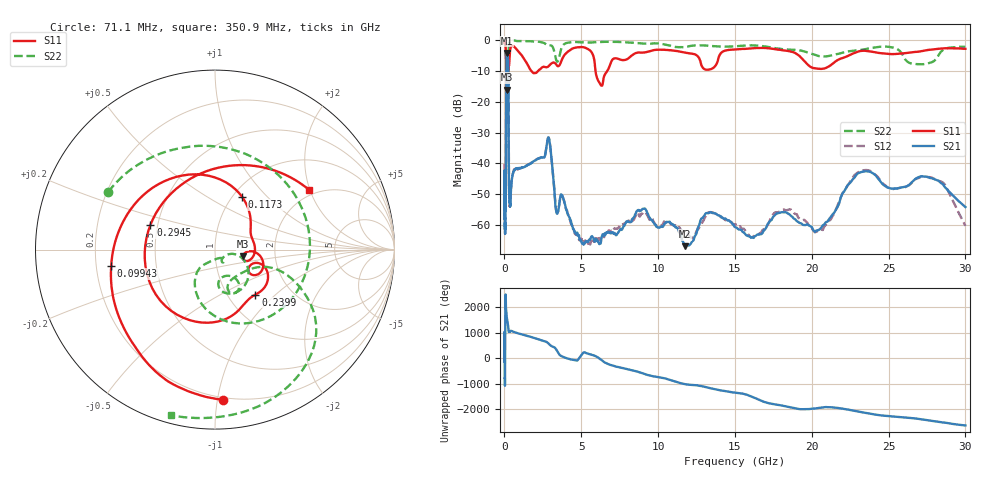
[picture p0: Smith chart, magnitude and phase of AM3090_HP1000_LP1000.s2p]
! Date/Time: Thu, Feb 28, 2019 2:02 PM
! Network Analyzer: Agilent Technologies E8364B Rev: A.07.50.67
! Sweep from 0.010 to 30.000 GHz, 1601 Points, Sweep Type: LOG
! Power Supply: 5.023 V, 0.002 A
# Hz S DB R 50
!freq MagS11 AngS11 MagS21 AngS21 MagS12 AngS12 MagS22 AngS22
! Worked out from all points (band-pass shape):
!   1601 points, 10 MHz to 30 GHz, reference 50 ohm
!   highest |S21| = -4.20 dB at 159.9 MHz (marker M1); lowest = -66.9 dB at 11.77 GHz (marker M2)
!   |S21| within 3 dB of the highest: 122.3 MHz to 242.5 MHz (120.2 MHz wide, 65.9 % of centre)
!   lowest |S11| = -16.0 dB at 152.9 MHz (marker M3), VSWR 1.37, Z = 67.9 - j5.19 ohm
!   |S11| at or under -10 dB: 118 MHz to 223 MHz (105 MHz wide, 61.6 % of centre); 1.745 GHz to 2.193 GHz (447.8 MHz wide, 22.7 % of centre); 5.925 GHz to 6.695 GHz (770.7 MHz wide, 12.2 % of centre)
!   |S22| runs from -25.7 to -0.1 dB; largest |S21 - S12| = 0.0097
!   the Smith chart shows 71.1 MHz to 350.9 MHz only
!   S11 on the Smith chart (normalised r, x): 71.1 MHz: 0.19, -1.04; 99.43 MHz: 0.26, -0.07; 117.3 MHz: 1.10, +0.73; 239.9 MHz: 1.34, -0.76; 294.5 MHz: 0.46, +0.15; 350.9 MHz: 1.83, +1.98
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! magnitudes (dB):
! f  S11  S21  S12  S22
! 10 MHz  -0.2  -42.4  -40.2  -0.6
! 38.04 MHz  -0.5  -59.0  -58.6  -1.5
! 71.1 MHz  -1.5  -54.5  -52.4  -3.4
! 86.86 MHz  -2.8  -53.2  -51.8  -4.9
! 99.43 MHz  -4.7  -33.7  -33.8  -5.5
! 117.3 MHz  -9.6  -10.1  -10.1  -12.5
! 144.7 MHz  -14.6  -4.4  -4.4  -23.9
! 152.9 MHz  -16.0  -4.2  -4.2  -21.3
! 159.9 MHz  -14.9  -4.2  -4.1  -16.6
! 239.9 MHz  -9.4  -6.9  -6.8  -13.5
! 294.5 MHz  -8.3  -48.1  -47.8  -1.2
! 350.9 MHz  -4.1  -52.7  -53.9  -0.4
! 550.5 MHz  -2.0  -43.3  -43.3  -0.2
! 2.084 GHz  -10.6  -38.8  -38.7  -0.5
! 2.884 GHz  -8.4  -31.8  -31.7  -1.8
! 3.402 GHz  -8.2  -56.2  -55.7  -6.9
! 5.077 GHz  -2.3  -66.2  -64.7  -0.7
! 7.926 GHz  -6.3  -58.9  -59.1  -0.7
! 11.77 GHz  -4.1  -66.9  -62.2  -2.2
! 20.51 GHz  -9.3  -61.5  -61.6  -5.2
! 23.48 GHz  -3.5  -42.6  -42.2  -2.9
! 30 GHz  -2.8  -54.2  -60.3  -2.2
